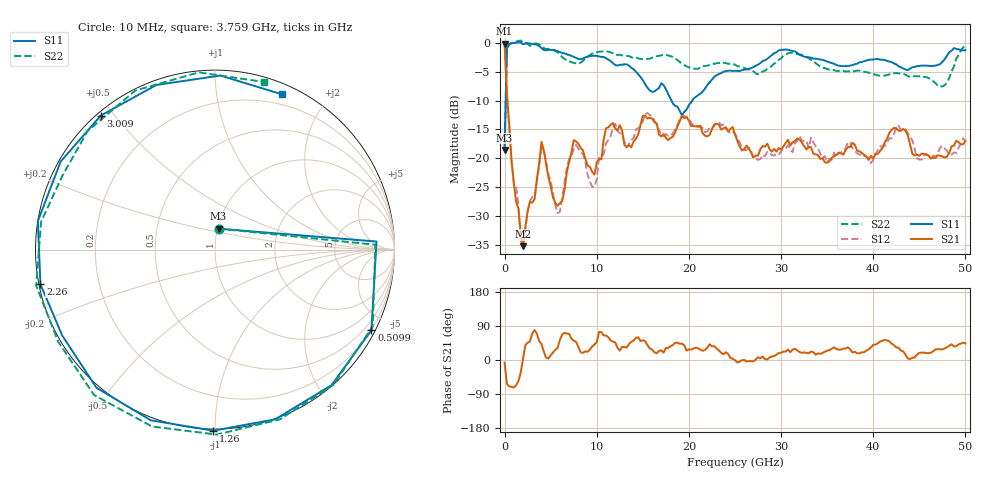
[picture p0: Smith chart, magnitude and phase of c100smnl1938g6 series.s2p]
! 10/28/2024 7:14:47 AM
! D:\C100SMNL1938G6 SERIES.S2P
! CHANNEL.1
! TR.MEASUREMENT
! CORRECTED.DATA
# GHZ S RI R 50.0
! FREQ.GHZ  S11RE  S11IM  S21RE  S21IM  S12RE  S12IM  S22RE  S22IM
!; PortSelection: Port_12
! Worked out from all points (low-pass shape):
!   201 points, 10 MHz to 50 GHz, reference 50 ohm
!   highest |S21| = -0.10 dB at 10 MHz (marker M1); lowest = -35.3 dB at 2.01 GHz (marker M2)
!   |S21| within 3 dB of the highest: start of sweep to 97.37 MHz
!   lowest |S11| = -18.6 dB at 10 MHz (marker M3), VSWR 1.27, Z = 50.6 + j12 ohm
!   |S11| at or under -10 dB: start of sweep to 131.1 MHz; 18.11 GHz to 20.36 GHz (2.25 GHz wide, 11.7 % of centre)
!   |S22| runs from -18.5 to 0.5 dB; largest |S21 - S12| = 0.064
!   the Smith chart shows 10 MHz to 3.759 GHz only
!   S11 on the Smith chart (normalised r, x): 10 MHz: 1.01, +0.24; 509.9 MHz: 0.18, -4.12; 1.26 GHz: -0.01, -0.99; 2.26 GHz: 0.00, -0.10; 3.009 GHz: 0.01, +0.46; 3.759 GHz: 0.10, +1.52
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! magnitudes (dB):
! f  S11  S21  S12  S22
! 10 MHz  -18.6  -0.1  -0.1  -18.5
! 259.9 MHz  -0.9  -8.7  -9.1  -1.0
! 509.9 MHz  -0.2  -14.3  -14.5  -0.2
! 1.26 GHz  0.1  -27.6  -24.9  0.3
! 2.01 GHz  -0.2  -35.3  -35.2  0.1
! 2.26 GHz  -0.1  -32.0  -32.4  0.1
! 3.009 GHz  -0.2  -27.7  -26.7  -0.3
! 3.759 GHz  -0.5  -20.9  -21.4  -0.2
! 4.259 GHz  -1.2  -18.6  -18.4  -0.9
! 5.759 GHz  -1.4  -28.3  -29.5  -1.6
! 7.508 GHz  -2.4  -16.8  -18.4  -3.4
! 8.508 GHz  -2.7  -18.6  -19.2  -3.1
! 9.758 GHz  -2.2  -22.8  -25.0  -1.6
! 12.01 GHz  -3.8  -14.8  -14.0  -2.0
! 16.76 GHz  -7.8  -15.9  -15.1  -2.2
! 19.26 GHz  -12.6  -12.5  -12.9  -3.5
! 25 GHz  -4.8  -15.9  -15.7  -3.7
! 33.5 GHz  -2.7  -19.2  -17.3  -3.2
! 39.75 GHz  -2.9  -19.6  -20.8  -5.3
! 41.75 GHz  -3.2  -15.6  -16.5  -5.4
! 47.5 GHz  -3.3  -19.7  -17.8  -7.5
! 50 GHz  -1.2  -17.0  -17.1  -0.5
